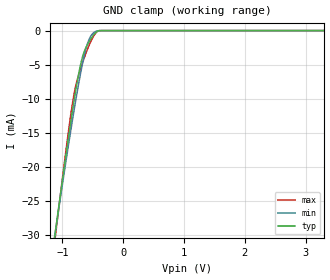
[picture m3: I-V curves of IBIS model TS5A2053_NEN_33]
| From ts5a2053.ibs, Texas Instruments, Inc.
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[Model]   TS5A2053_NEN_33
Model_type  Input
Vinl=0.8
Vinh=2.0
| variable   typ   min   max
C_comp   3.31pF   2.76pF   4.30pF
[Temperature Range]   40   100   -40
| Ambient temperature   25   85   -40
[Voltage range]   3.3   3   3.6
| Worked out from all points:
|   GND clamp passes 1 mA (typ) near -0.52 V on its own axis
[GND Clamp]
| TS5A2053_NEN_33
|   Voltage   I(typ)   I(min)   I(max)
-5.5V     -348.1mA   -320.8mA   -389.9mA
-1.15V    -31.74mA   -31.56mA   -32.72mA
-1.11V    -29.1mA    -29.13mA   -29.74mA
-895mV    -15.37mA   -16.48mA   -14.42mA
-840mV    -12.09mA   -13.41mA   -10.99mA
-800mV    -9.814mA   -11.25mA   -8.913mA
-725mV    -5.999mA   -7.404mA   -6.269mA
-660mV    -3.579mA   -4.449mA   -4.491mA
-575mV    -1.843mA   -1.604mA   -2.457mA
-485mV    -638.7uA   -307.3uA   -791.6uA
-390mV    -8.587uA   -16.56uA   -7.146uA
3.3V      166.6pA    583.6pA    1.325nA
